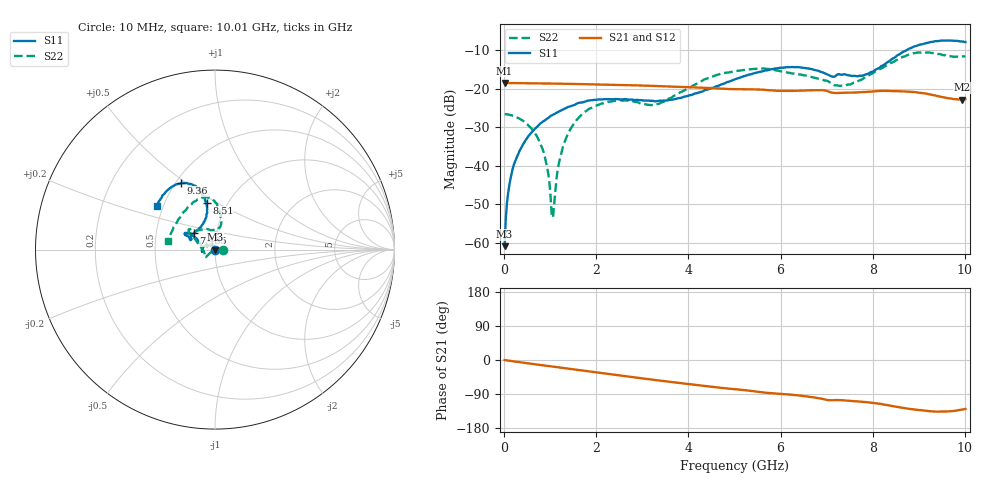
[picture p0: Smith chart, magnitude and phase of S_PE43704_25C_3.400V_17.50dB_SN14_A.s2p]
! Device ID: PE43704
! Dir: z:\PE43704\PE43704_Char_1_20130516\PE43704\AMB\3p400V\17p50dB
! Serial: 14
! Insertion: A
! Impedance: 50 ohm
! Temp: Amb
! VDD: 3.400V
! Attenuation Step: 17.50dB
! IDD: 1.140585e-01mA
#  Hz  S  RI  R  50
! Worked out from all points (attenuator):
!   401 points, 10 MHz to 10.01 GHz, reference 50 ohm
!   highest |S21| = -18.47 dB at 10 MHz (marker M1); lowest = -22.8 dB at 9.935 GHz (marker M2)
!   lowest |S11| = -60.8 dB at 10 MHz (marker M3), VSWR 1.00, Z = 50.1 + j0.0433 ohm
!   |S11| at or under -10 dB: start of sweep to 8.726 GHz
!   |S22| runs from -53.3 to -10.5 dB; largest |S21 - S12| = 0.0012
!   S11 on the Smith chart (normalised r, x): 10 MHz: 1.00, +0.00; 7.485 GHz: 0.78, +0.15; 8.51 GHz: 0.80, +0.45; 9.36 GHz: 0.53, +0.48; 10.01 GHz: 0.46, +0.27
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1e7  0.0008 0.000432  0.1192 -0.00035  0.1193 -0.000414  0.047 3.56e-05
1.1e8  0.000739 0.00545  0.1189 -0.00408  0.1188 -0.00406  0.046 0.00119
2.6e8  -0.00137 0.0123  0.1183 -0.00931  0.1183 -0.00924  0.0428 0.00377
5.6e8  -0.0104 0.0236  0.1165 -0.0194  0.1166 -0.0194  0.0315 0.00619
7.85e8  -0.0211 0.0287  0.1147 -0.0269  0.1146 -0.0268  0.0189 0.00437
9.1e8  -0.0277 0.0291  0.1134 -0.0308  0.1133 -0.0308  0.0108 0.00219
1.01e9  -0.0333 0.0296  0.1123 -0.034  0.1122 -0.0339  0.00383 -0.00017
1.06e9  -0.0361 0.0288  0.1117 -0.0356  0.1117 -0.0354  0.000276 -0.00216
1.185e9  -0.0426 0.0273  0.1099 -0.0395  0.11 -0.0395  -0.00848 -0.00643
1.285e9  -0.0478 0.0256  0.1085 -0.0424  0.1085 -0.0424  -0.0155 -0.0102
1.685e9  -0.0651 0.0141  0.102 -0.0539  0.102 -0.0538  -0.0377 -0.0277
2.36e9  -0.0732 -0.00505  0.0883 -0.0703  0.0883 -0.0703  -0.0545 -0.0427
3.36e9  -0.0702 -0.00216  0.0636 -0.0879  0.0637 -0.0879  -0.0637 -0.00721
5.01e9  -0.1129 0.0699  0.0223 -0.0968  0.0223 -0.0969  -0.1413 0.0926
5.96e9  -0.1612 0.0931  0.00164 -0.0943  0.00178 -0.0943  -0.1329 0.108
6.685e9  -0.162 0.0791  -0.0137 -0.0949  -0.0136 -0.0949  -0.092 0.1077
7.485e9  -0.1176 0.0934  -0.0275 -0.0852  -0.0274 -0.0853  0.00798 0.1138
8.36e9  -0.044 0.2254  -0.047 -0.0813  -0.047 -0.0816  0.0282 0.2084
8.51e9  -0.047 0.2603  -0.0513 -0.0778  -0.0511 -0.0787  0.0188 0.2349
9.36e9  -0.1882 0.3714  -0.0589 -0.0568  -0.059 -0.0565  -0.1243 0.2621
9.935e9  -0.3115 0.2704  -0.0474 -0.0551  -0.0484 -0.0551  -0.2492 0.0835
1.001e10  -0.3233 0.2439  -0.0466 -0.057  -0.0478 -0.0572  -0.2605 0.0505
